(* Logix 5000 AddOnInstructionDefinition export AMCI_NXFE2_Program_Blend_Move; software revision 20.03 *)

ADD_ON_INSTRUCTION AMCI_NXFE2_Program_Blend_Move   (* revision 1.0, ExecuteEnableInFalse *)
VAR_INPUT
   Status_Bits_MSW : INT; {required}
        .9   // Set when invalid profile error
   Status_Bits_LSW : INT; {required}
        .9   // The NXFE2 module sets this bit to Acknowledge the receipt of a blend move programming block
   Number_of_Segments : INT; {required}
   Final_Move_Deceleration : INT; {required}
   Acceleration_Type_segments_9_to_16 : INT;
   Acceleration_Type_segments_1_to_8 : INT;
   Segment_1_Distance : DINT; {required}
   Segment_1_Programmed_Speed : DINT; {required}
   Segment_1_Acceleration_Deceleration : INT; {required}
   Segment_2_Distance : DINT; {required}
   Segment_2_Programmed_Speed : DINT; {required}
   Segment_2_Acceleration_Deceleration : INT; {required}
   Segment_3_Distance : DINT; {required}
   Segment_3_Programmed_Speed : DINT; {required}
   Segment_3_Acceleration_Deceleration : INT; {required}
   Segment_4_Distance : DINT; {required}
   Segment_4_Programmed_Speed : DINT; {required}
   Segment_4_Acceleration_Deceleration : INT; {required}
   Segment_5_Distance : DINT; {required}
   Segment_5_Programmed_Speed : DINT; {required}
   Segment_5_Acceleration_Deceleration : INT; {required}
   Segment_6_Distance : DINT; {required}
   Segment_6_Programmed_Speed : DINT; {required}
   Segment_6_Acceleration_Deceleration : INT; {required}
   Segment_7_Distance : DINT; {required}
   Segment_7_Programmed_Speed : DINT; {required}
   Segment_7_Acceleration_Deceleration : INT; {required}
   Segment_8_Distance : DINT; {required}
   Segment_8_Programmed_Speed : DINT; {required}
   Segment_8_Acceleration_Deceleration : INT; {required}
   Segment_9_Distance : DINT; {required}
   Segment_9_Programmed_Speed : DINT; {required}
   Segment_9_Acceleration_Deceleration : INT; {required}
   Segment_10_Distance : DINT; {required}
   Segment_10_Programmed_Speed : DINT; {required}
   Segment_10_Acceleration_Deceleration : INT; {required}
   Segment_11_Distance : DINT; {required}
   Segment_11_Programmed_Speed : DINT; {required}
   Segment_11_Acceleration_Deceleration : INT; {required}
   Segment_12_Distance : DINT; {required}
   Segment_12_Programmed_Speed : DINT; {required}
   Segment_12_Acceleration_Deceleration : INT; {required}
   Segment_13_Distance : DINT; {required}
   Segment_13_Programmed_Speed : DINT; {required}
   Segment_13_Acceleration_Deceleration : INT; {required}
   Segment_14_Distance : DINT; {required}
   Segment_14_Programmed_Speed : DINT; {required}
   Segment_14_Acceleration_Deceleration : INT; {required}
   Segment_15_Distance : DINT; {required}
   Segment_15_Programmed_Speed : DINT; {required}
   Segment_15_Acceleration_Deceleration : INT; {required}
   Segment_16_Distance : DINT; {required}
   Segment_16_Programmed_Speed : DINT; {required}
   Segment_16_Acceleration_Deceleration : INT; {required}
END_VAR
VAR_IN_OUT
   NXFE2_output_data : _000A:NXFE2_0986AEB4:O:0; {required}
END_VAR
VAR_OUTPUT
   Blend_Move_Programmed : BOOL; {access Read Only, visible}
END_VAR
VAR
   command_data_block : INT[10];
   Blend_Move_setup : INT[10] := ([1] := -32640);
   Blend_Move_counter : COUNTER;
   Programmed_Speed : DINT;
   Distance : DINT;
END_VAR

ROUTINE EnableInFalse   (* ladder *)
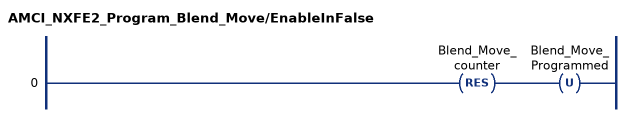
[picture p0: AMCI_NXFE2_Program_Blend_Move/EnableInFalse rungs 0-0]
   0: RES(Blend_Move_counter)OTU(Blend_Move_Programmed);
END_ROUTINE

ROUTINE Logic   (* ladder *)
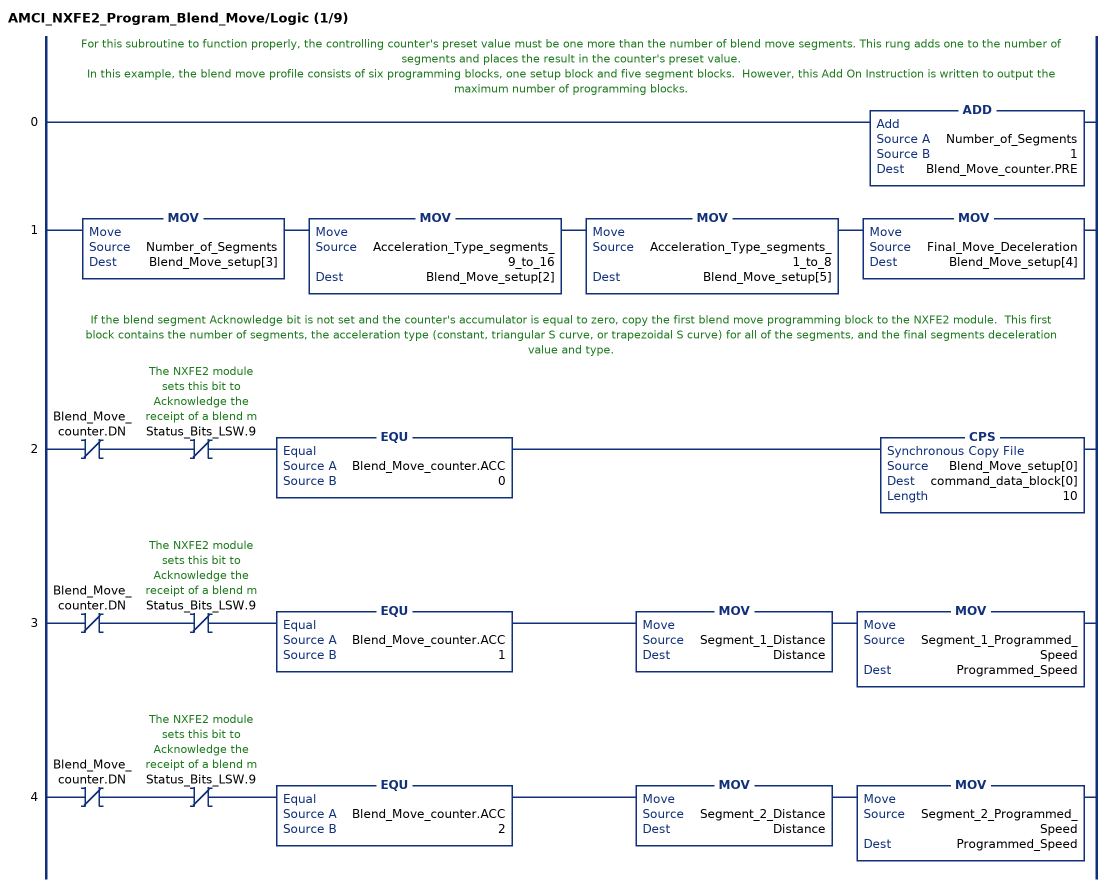
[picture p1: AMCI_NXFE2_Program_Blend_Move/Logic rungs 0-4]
   // For this subroutine to function properly, the controlling counter's preset value must be one more than the number of blend move segments. This rung adds one to the number of segments and places the result in the counter's preset value.
   // In this example, the blend move profile consists of six programming blocks, one setup block and five segment blocks.  However, this Add On Instruction is written to output the maximum number of programming blocks.
   0: ADD(Number_of_Segments,1,Blend_Move_counter.PRE);
   1: MOV(Number_of_Segments,Blend_Move_setup[3])MOV(Acceleration_Type_segments_9_to_16,Blend_Move_setup[2])MOV(Acceleration_Type_segments_1_to_8,Blend_Move_setup[5])MOV(Final_Move_Deceleration,Blend_Move_setup[4]);
   // If the blend segment Acknowledge bit is not set and the counter's accumulator is equal to zero, copy the first blend move programming block to the NXFE2 module.  This first block contains the number of segments, the acceleration type (constant, triangular S curve, or trapezoidal S curve) for all of the segments, and the final segments deceleration value and type.
   2: XIO(Blend_Move_counter.DN)XIO(Status_Bits_LSW.9)EQU(Blend_Move_counter.ACC,0)CPS(Blend_Move_setup[0],command_data_block[0],10);
   3: XIO(Blend_Move_counter.DN)XIO(Status_Bits_LSW.9)EQU(Blend_Move_counter.ACC,1)MOV(Segment_1_Distance,Distance)MOV(Segment_1_Programmed_Speed,Programmed_Speed);
   4: XIO(Blend_Move_counter.DN)XIO(Status_Bits_LSW.9)EQU(Blend_Move_counter.ACC,2)MOV(Segment_2_Distance,Distance)MOV(Segment_2_Programmed_Speed,Programmed_Speed);
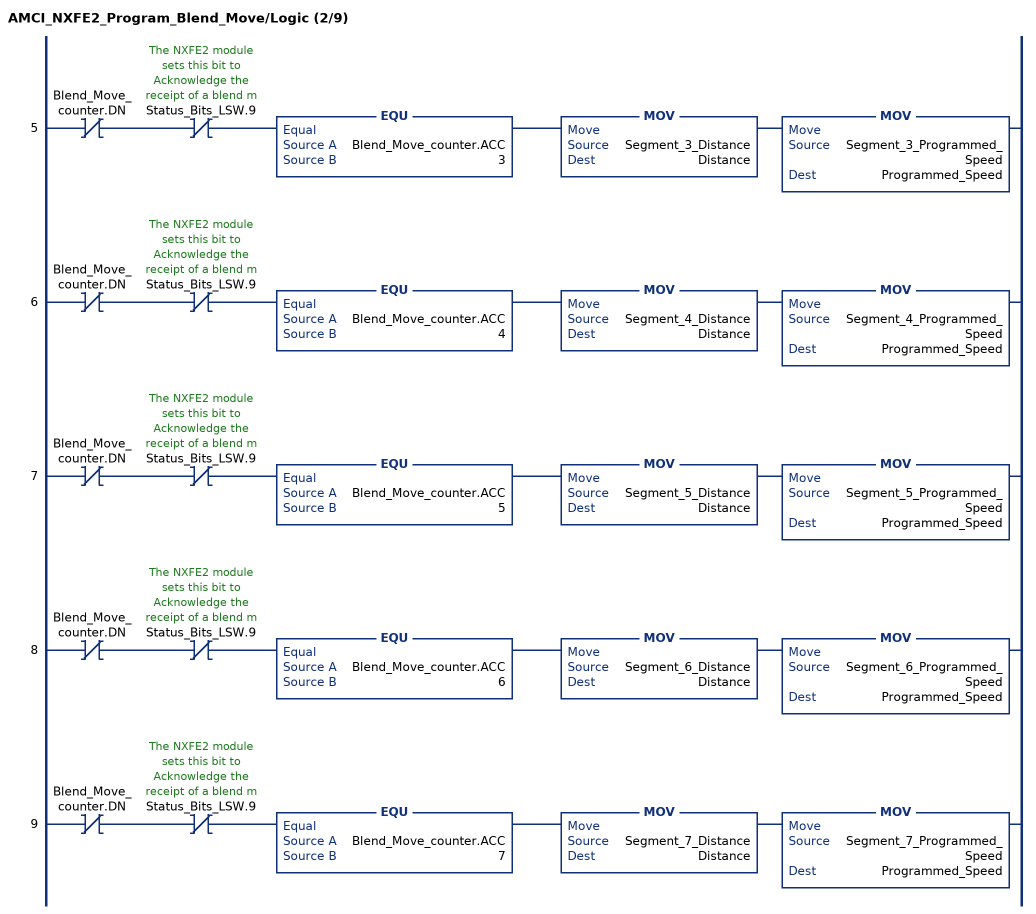
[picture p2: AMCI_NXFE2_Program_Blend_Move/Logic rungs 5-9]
   5: XIO(Blend_Move_counter.DN)XIO(Status_Bits_LSW.9)EQU(Blend_Move_counter.ACC,3)MOV(Segment_3_Distance,Distance)MOV(Segment_3_Programmed_Speed,Programmed_Speed);
   6: XIO(Blend_Move_counter.DN)XIO(Status_Bits_LSW.9)EQU(Blend_Move_counter.ACC,4)MOV(Segment_4_Distance,Distance)MOV(Segment_4_Programmed_Speed,Programmed_Speed);
   7: XIO(Blend_Move_counter.DN)XIO(Status_Bits_LSW.9)EQU(Blend_Move_counter.ACC,5)MOV(Segment_5_Distance,Distance)MOV(Segment_5_Programmed_Speed,Programmed_Speed);
   8: XIO(Blend_Move_counter.DN)XIO(Status_Bits_LSW.9)EQU(Blend_Move_counter.ACC,6)MOV(Segment_6_Distance,Distance)MOV(Segment_6_Programmed_Speed,Programmed_Speed);
   9: XIO(Blend_Move_counter.DN)XIO(Status_Bits_LSW.9)EQU(Blend_Move_counter.ACC,7)MOV(Segment_7_Distance,Distance)MOV(Segment_7_Programmed_Speed,Programmed_Speed);
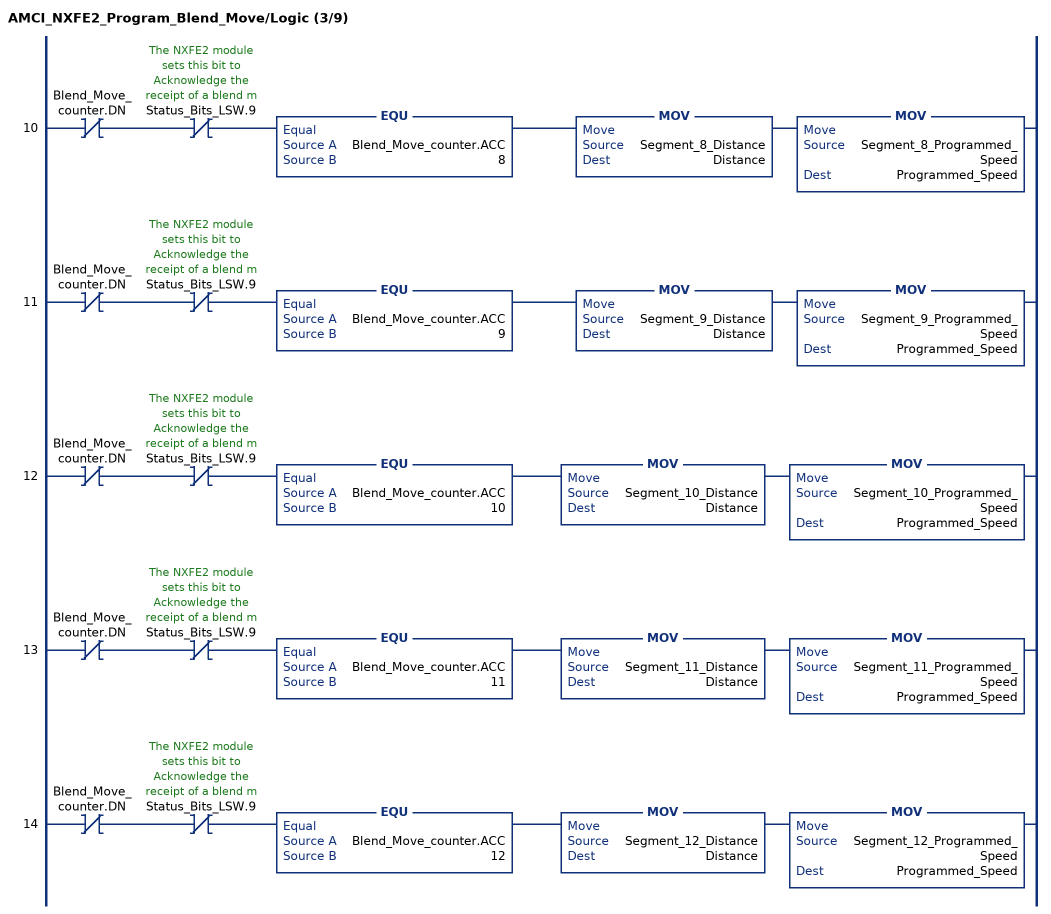
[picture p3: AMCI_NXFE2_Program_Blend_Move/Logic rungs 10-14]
   10: XIO(Blend_Move_counter.DN)XIO(Status_Bits_LSW.9)EQU(Blend_Move_counter.ACC,8)MOV(Segment_8_Distance,Distance)MOV(Segment_8_Programmed_Speed,Programmed_Speed);
   11: XIO(Blend_Move_counter.DN)XIO(Status_Bits_LSW.9)EQU(Blend_Move_counter.ACC,9)MOV(Segment_9_Distance,Distance)MOV(Segment_9_Programmed_Speed,Programmed_Speed);
   12: XIO(Blend_Move_counter.DN)XIO(Status_Bits_LSW.9)EQU(Blend_Move_counter.ACC,10)MOV(Segment_10_Distance,Distance)MOV(Segment_10_Programmed_Speed,Programmed_Speed);
   13: XIO(Blend_Move_counter.DN)XIO(Status_Bits_LSW.9)EQU(Blend_Move_counter.ACC,11)MOV(Segment_11_Distance,Distance)MOV(Segment_11_Programmed_Speed,Programmed_Speed);
   14: XIO(Blend_Move_counter.DN)XIO(Status_Bits_LSW.9)EQU(Blend_Move_counter.ACC,12)MOV(Segment_12_Distance,Distance)MOV(Segment_12_Programmed_Speed,Programmed_Speed);
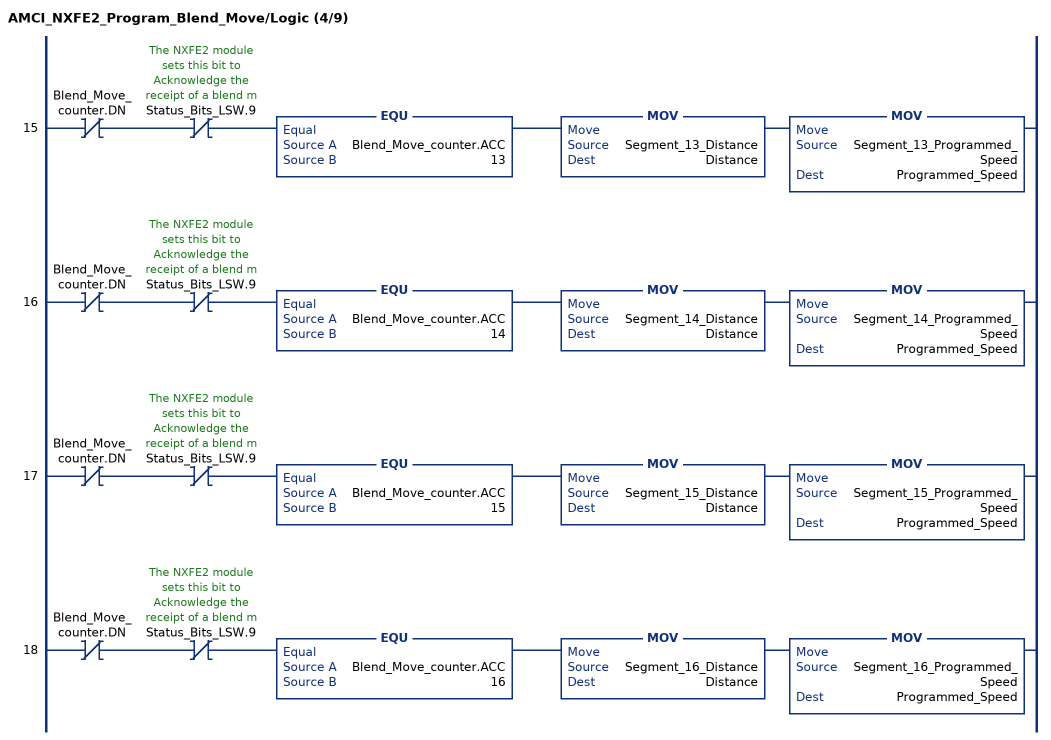
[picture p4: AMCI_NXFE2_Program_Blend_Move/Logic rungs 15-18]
   15: XIO(Blend_Move_counter.DN)XIO(Status_Bits_LSW.9)EQU(Blend_Move_counter.ACC,13)MOV(Segment_13_Distance,Distance)MOV(Segment_13_Programmed_Speed,Programmed_Speed);
   16: XIO(Blend_Move_counter.DN)XIO(Status_Bits_LSW.9)EQU(Blend_Move_counter.ACC,14)MOV(Segment_14_Distance,Distance)MOV(Segment_14_Programmed_Speed,Programmed_Speed);
   17: XIO(Blend_Move_counter.DN)XIO(Status_Bits_LSW.9)EQU(Blend_Move_counter.ACC,15)MOV(Segment_15_Distance,Distance)MOV(Segment_15_Programmed_Speed,Programmed_Speed);
   18: XIO(Blend_Move_counter.DN)XIO(Status_Bits_LSW.9)EQU(Blend_Move_counter.ACC,16)MOV(Segment_16_Distance,Distance)MOV(Segment_16_Programmed_Speed,Programmed_Speed);
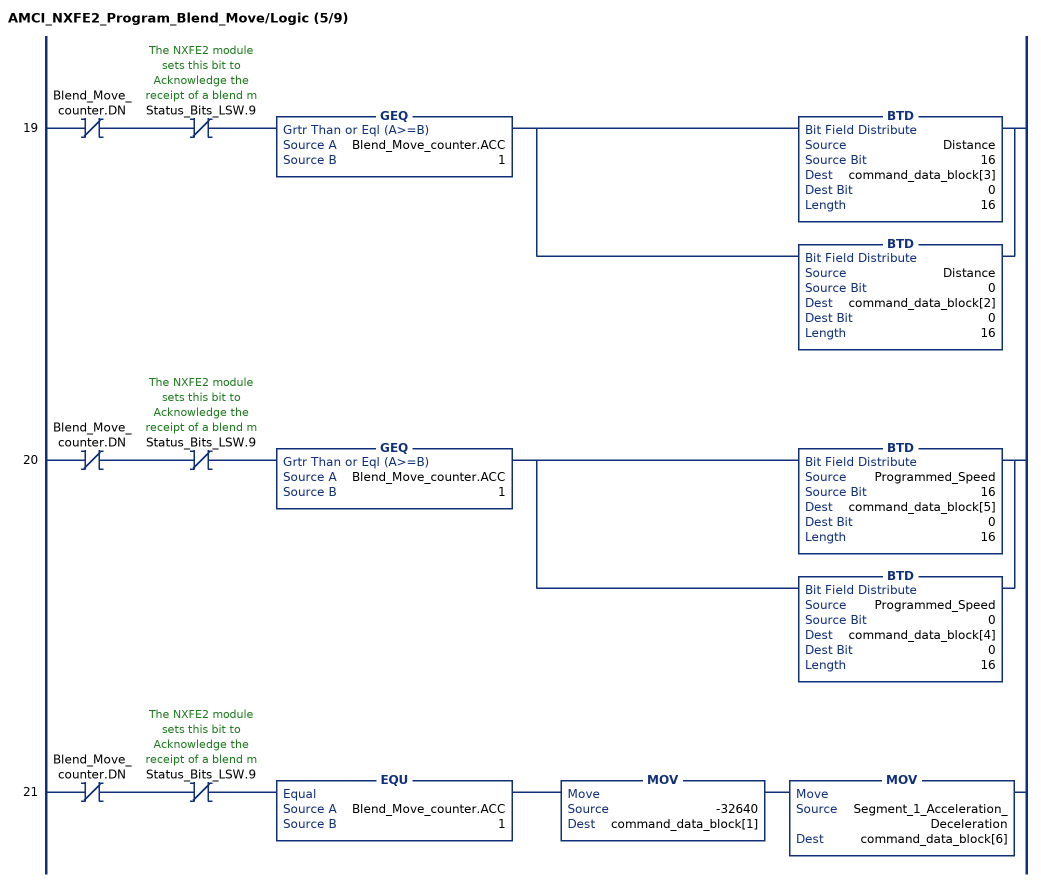
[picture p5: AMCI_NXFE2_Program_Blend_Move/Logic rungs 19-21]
   19: XIO(Blend_Move_counter.DN)XIO(Status_Bits_LSW.9)GEQ(Blend_Move_counter.ACC,1)[BTD(Distance,16,command_data_block[3],0,16) ,BTD(Distance,0,command_data_block[2],0,16) ];
   20: XIO(Blend_Move_counter.DN)XIO(Status_Bits_LSW.9)GEQ(Blend_Move_counter.ACC,1)[BTD(Programmed_Speed,16,command_data_block[5],0,16) ,BTD(Programmed_Speed,0,command_data_block[4],0,16) ];
   21: XIO(Blend_Move_counter.DN)XIO(Status_Bits_LSW.9)EQU(Blend_Move_counter.ACC,1)MOV(-32640,command_data_block[1])MOV(Segment_1_Acceleration_Deceleration,command_data_block[6]);
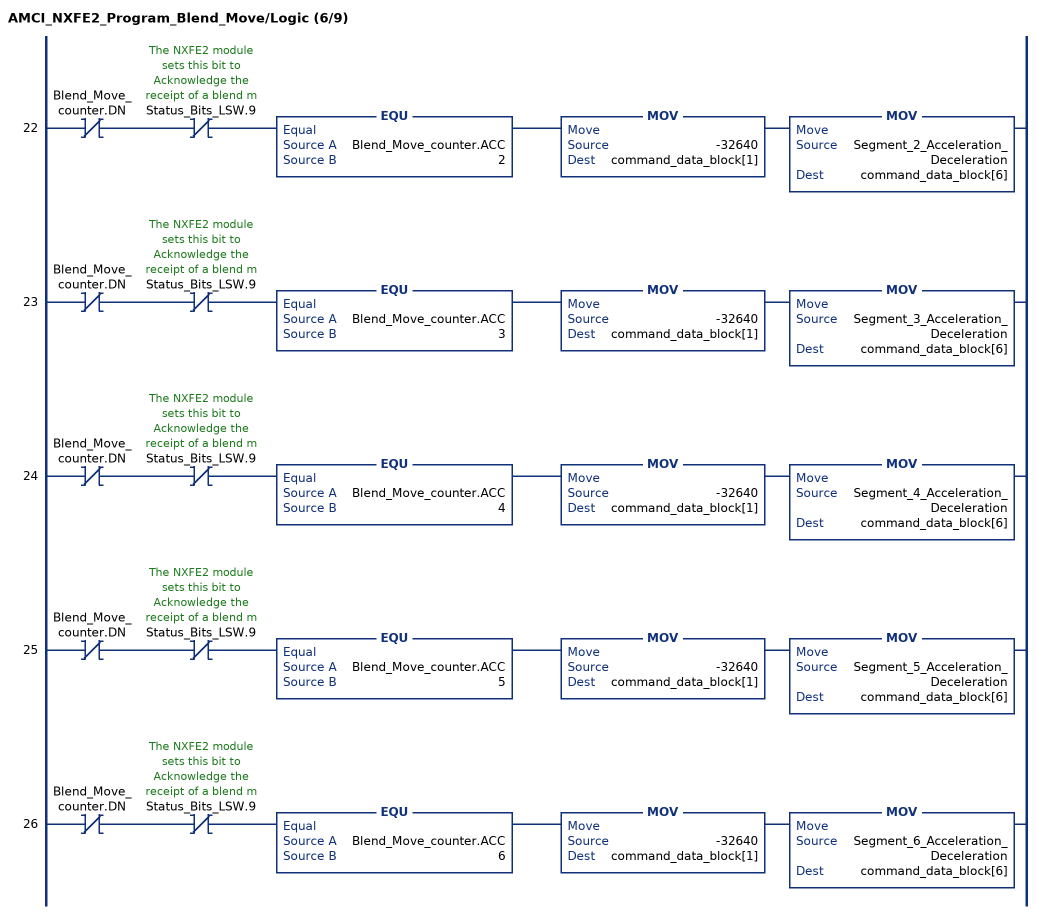
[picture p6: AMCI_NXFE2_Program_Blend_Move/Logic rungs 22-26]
   22: XIO(Blend_Move_counter.DN)XIO(Status_Bits_LSW.9)EQU(Blend_Move_counter.ACC,2)MOV(-32640,command_data_block[1])MOV(Segment_2_Acceleration_Deceleration,command_data_block[6]);
   23: XIO(Blend_Move_counter.DN)XIO(Status_Bits_LSW.9)EQU(Blend_Move_counter.ACC,3)MOV(-32640,command_data_block[1])MOV(Segment_3_Acceleration_Deceleration,command_data_block[6]);
   24: XIO(Blend_Move_counter.DN)XIO(Status_Bits_LSW.9)EQU(Blend_Move_counter.ACC,4)MOV(-32640,command_data_block[1])MOV(Segment_4_Acceleration_Deceleration,command_data_block[6]);
   25: XIO(Blend_Move_counter.DN)XIO(Status_Bits_LSW.9)EQU(Blend_Move_counter.ACC,5)MOV(-32640,command_data_block[1])MOV(Segment_5_Acceleration_Deceleration,command_data_block[6]);
   26: XIO(Blend_Move_counter.DN)XIO(Status_Bits_LSW.9)EQU(Blend_Move_counter.ACC,6)MOV(-32640,command_data_block[1])MOV(Segment_6_Acceleration_Deceleration,command_data_block[6]);
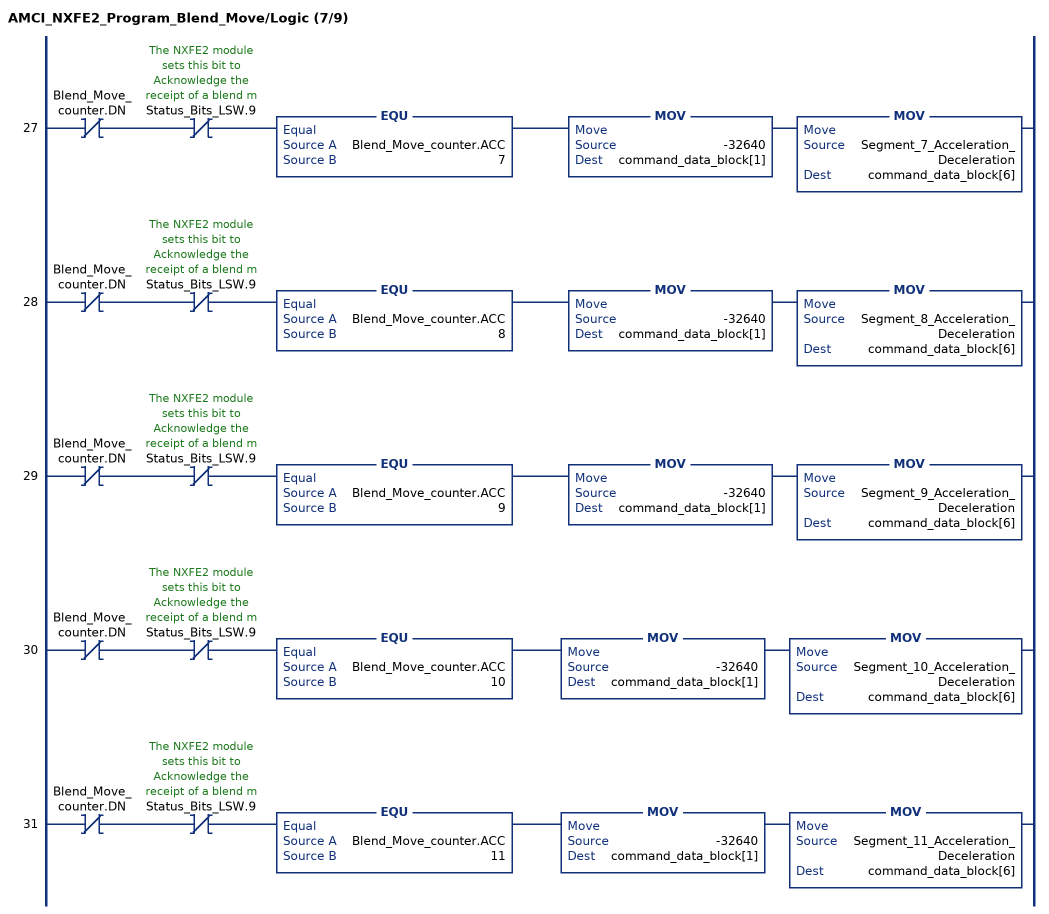
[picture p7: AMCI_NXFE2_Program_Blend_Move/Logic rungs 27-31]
   27: XIO(Blend_Move_counter.DN)XIO(Status_Bits_LSW.9)EQU(Blend_Move_counter.ACC,7)MOV(-32640,command_data_block[1])MOV(Segment_7_Acceleration_Deceleration,command_data_block[6]);
   28: XIO(Blend_Move_counter.DN)XIO(Status_Bits_LSW.9)EQU(Blend_Move_counter.ACC,8)MOV(-32640,command_data_block[1])MOV(Segment_8_Acceleration_Deceleration,command_data_block[6]);
   29: XIO(Blend_Move_counter.DN)XIO(Status_Bits_LSW.9)EQU(Blend_Move_counter.ACC,9)MOV(-32640,command_data_block[1])MOV(Segment_9_Acceleration_Deceleration,command_data_block[6]);
   30: XIO(Blend_Move_counter.DN)XIO(Status_Bits_LSW.9)EQU(Blend_Move_counter.ACC,10)MOV(-32640,command_data_block[1])MOV(Segment_10_Acceleration_Deceleration,command_data_block[6]);
   31: XIO(Blend_Move_counter.DN)XIO(Status_Bits_LSW.9)EQU(Blend_Move_counter.ACC,11)MOV(-32640,command_data_block[1])MOV(Segment_11_Acceleration_Deceleration,command_data_block[6]);
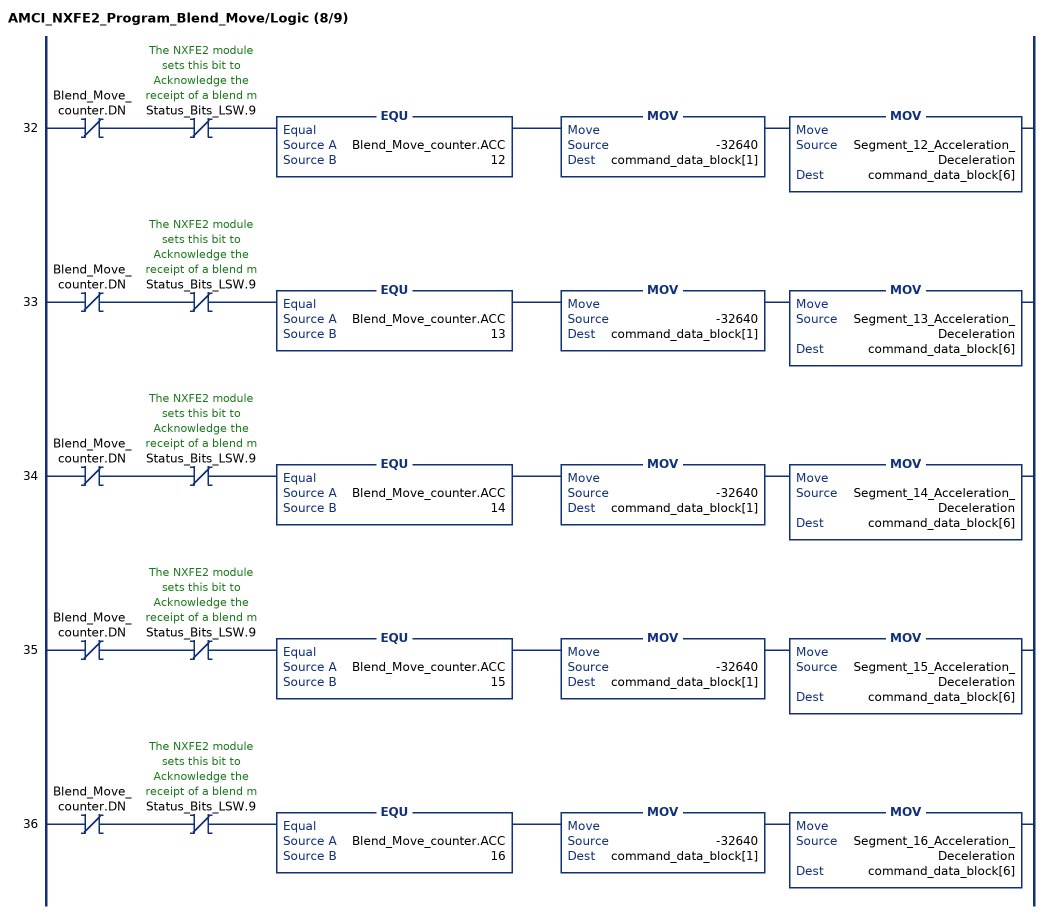
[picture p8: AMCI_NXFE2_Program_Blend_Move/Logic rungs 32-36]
   32: XIO(Blend_Move_counter.DN)XIO(Status_Bits_LSW.9)EQU(Blend_Move_counter.ACC,12)MOV(-32640,command_data_block[1])MOV(Segment_12_Acceleration_Deceleration,command_data_block[6]);
   33: XIO(Blend_Move_counter.DN)XIO(Status_Bits_LSW.9)EQU(Blend_Move_counter.ACC,13)MOV(-32640,command_data_block[1])MOV(Segment_13_Acceleration_Deceleration,command_data_block[6]);
   34: XIO(Blend_Move_counter.DN)XIO(Status_Bits_LSW.9)EQU(Blend_Move_counter.ACC,14)MOV(-32640,command_data_block[1])MOV(Segment_14_Acceleration_Deceleration,command_data_block[6]);
   35: XIO(Blend_Move_counter.DN)XIO(Status_Bits_LSW.9)EQU(Blend_Move_counter.ACC,15)MOV(-32640,command_data_block[1])MOV(Segment_15_Acceleration_Deceleration,command_data_block[6]);
   36: XIO(Blend_Move_counter.DN)XIO(Status_Bits_LSW.9)EQU(Blend_Move_counter.ACC,16)MOV(-32640,command_data_block[1])MOV(Segment_16_Acceleration_Deceleration,command_data_block[6]);
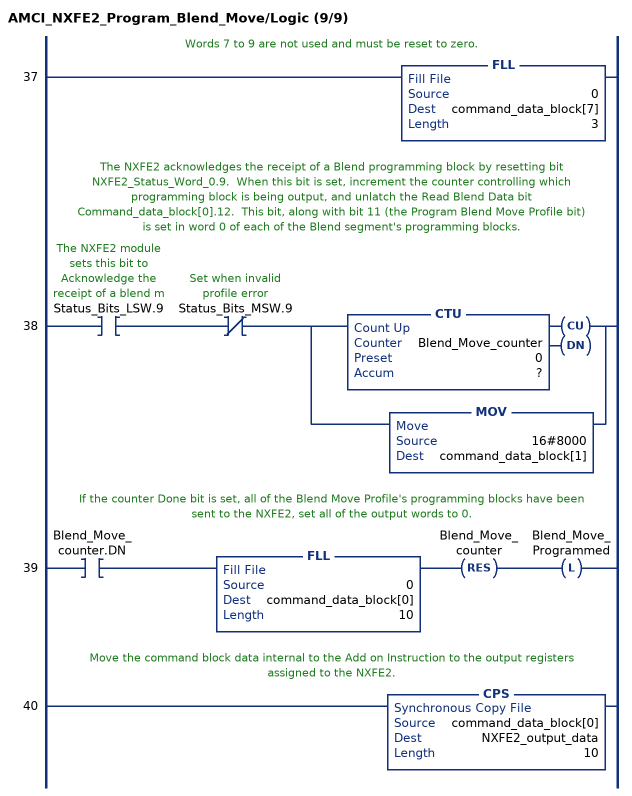
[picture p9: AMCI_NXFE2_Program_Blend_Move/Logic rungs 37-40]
   // Words 7 to 9 are not used and must be reset to zero.
   37: FLL(0,command_data_block[7],3);
   // The NXFE2 acknowledges the receipt of a Blend programming block by resetting bit NXFE2_Status_Word_0.9.  When this bit is set, increment the counter controlling which programming block is being output, and unlatch the Read Blend Data bit Command_data_block[0].12.  This bit, along with bit 11 (the Program Blend Move Profile bit)  is set in word 0 of each of the Blend segment's programming blocks.
   38: XIC(Status_Bits_LSW.9)XIO(Status_Bits_MSW.9)[CTU(Blend_Move_counter,?,?) ,MOV(16#8000,command_data_block[1]) ];
   // If the counter Done bit is set, all of the Blend Move Profile's programming blocks have been sent to the NXFE2, set all of the output words to 0.
   39: XIC(Blend_Move_counter.DN)FLL(0,command_data_block[0],10)RES(Blend_Move_counter)OTL(Blend_Move_Programmed);
   // Move the command block data internal to the Add on Instruction to the output registers assigned to the NXFE2.
   40: CPS(command_data_block[0],NXFE2_output_data,10);
END_ROUTINE
END_ADD_ON_INSTRUCTION
